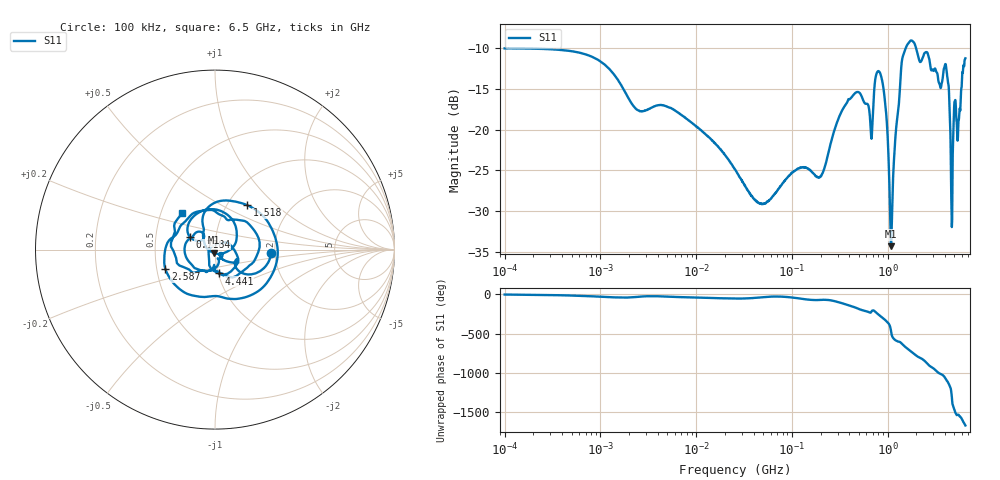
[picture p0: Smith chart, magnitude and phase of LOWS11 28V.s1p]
!Keysight Technologies,E5080B,MY59100498,A.17.05.10
!Date: Wednesday, August 30, 2023 18:48:44
!Correction: S11(C  1-Port  )
!S1P File: Measurement: S11:Log Frequency Sweep
# Hz S  dB  R 50
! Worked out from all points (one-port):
!   1601 points, 100 kHz to 6.5 GHz, reference 50 ohm
!   lowest |S11| = -34.3 dB at 1.089 GHz (marker M1), VSWR 1.04, Z = 49.2 - j1.75 ohm
!   |S11| at or under -10 dB: start of sweep to 1.554 GHz; 1.98 GHz to end of sweep
!   S11 on the Smith chart (normalised r, x): 100 kHz: 1.91, -0.07; 718.4 MHz: 0.75, +0.11; 1.518 GHz: 1.23, +0.67; 2.587 GHz: 0.56, -0.13; 4.441 GHz: 1.00, -0.27; 6.5 GHz: 0.64, +0.28
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100000  -10.08 -3.2
399589.6  -10.28 -12.7
1596718  -14.29 -41.4
2487396  -17.66 -32.0
6380321  -17.88 -34.5
2.54951e7  -24.87 -53.8
4.888947e7  -29.10 -37.7
1.018758e8  -25.24 -41.9
2.008454e8  -25.73 -71.0
4.070849e8  -16.24 -146.5
6.702952e8  -20.51 129.6
7.183677e8  -15.99 153.0
7.860529e8  -12.91 112.0
8.904243e8  -14.39 58.7
9.675956e8  -18.08 20.4
1.088507e9  -34.27 -113.4
1.330654e9  -15.90 115.5
1.517814e9  -10.30 54.2
1.626669e9  -9.54 26.1
2.002356e9  -10.21 -61.1
2.587259e9  -10.54 -158.3
3.274269e9  -13.04 97.8
4.115103e9  -12.66 -10.7
4.440884e9  -17.41 -81.3
4.759378e9  -26.61 47.0
5.065506e9  -16.44 -53.7
5.777982e9  -17.04 -122.9
6.5e9  -11.29 132.2
